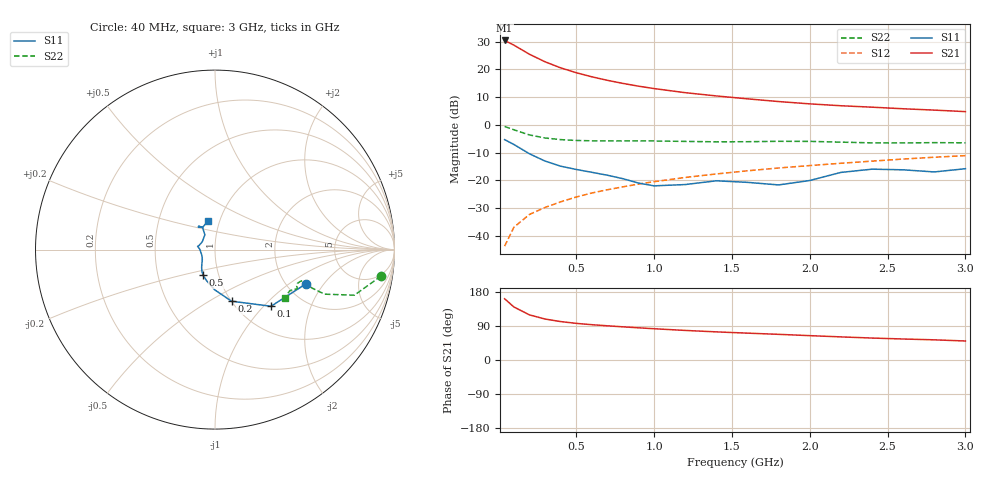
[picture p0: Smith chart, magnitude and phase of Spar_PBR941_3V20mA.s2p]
! Filename:  PBR941G.S2P  Version:  3.0
! NXP part #:  PBR941  Date: July 1998
! Bias condition:  Vce=3V, Ic=20mA
#  MHz  S  MA  R 50
! Freq  S11  S21  S12  S22
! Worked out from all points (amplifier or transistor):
!   21 points, 40 MHz to 3 GHz, reference 50 ohm
!   highest |S21| = 30.4 dB at 40 MHz (marker M1)
!   |S21| within 3 dB of that: start of sweep to 139.8 MHz
!   unconditionally stable (mu >= 1): 651.9 MHz to 2.236 GHz
!   at 300 MHz: K = 0.87, MSG = 26.2 dB, |S12| = -29.7 dB
!   at 1 GHz: K = 1.03, MAG = 15.7 dB, |S12| = -20.4 dB
!   at 3 GHz: K = 0.97, MSG = 7.9 dB, |S12| = -11.1 dB
!   S11 on the Smith chart (normalised r, x): 40 MHz: 2.55, -1.37; 100 MHz: 1.40, -1.10; 200 MHz: 1.00, -0.63; 500 MHz: 0.84, -0.25; 3 GHz: 0.88, +0.29
40  0.5433 -20.4  33.04 161.6  0.006582 81.4  0.9368 -9.1
100  0.444 -45.3  27.18 139.8  0.01444 74.7  0.8169 -18.1
200  0.3019 -72.3  18.64 119.0  0.02453 72.3  0.6591 -22.1
300  0.2233 -90.7  13.64 108.1  0.03277 74.9  0.5815 -21.6
400  0.181 -104.5  10.63 101.4  0.04127 76.0  0.5437 -20.7
500  0.1578 -114.9  8.688 96.7  0.05041 77.5  0.5252 -20.1
600  0.1404 -121.3  7.333 93.2  0.05953 78.1  0.5172 -19.8
700  0.1244 -126.7  6.342 90.2  0.06809 78.9  0.5151 -19.7
800  0.1077 -132.7  5.577 87.5  0.07686 79.3  0.5156 -19.6
900  0.0899 -142.0  4.975 85.0  0.08615 79.5  0.5151 -19.7
1000  0.08006 -155.2  4.504 82.5  0.0952 79.5  0.5138 -19.9
1200  0.08452 178.8  3.799 78.0  0.1133 79.3  0.5049 -20.7
1400  0.09872 169.3  3.319 74.2  0.1311 79.0  0.4961 -22.4
1600  0.09256 166.4  2.943 70.9  0.1494 78.8  0.4984 -24.1
1800  0.0832 148.7  2.631 67.7  0.1678 78.4  0.5067 -25.2
2000  0.09993 124.4  2.39 64.3  0.1855 77.5  0.5052 -25.9
2200  0.1397 119.4  2.211 61.0  0.204 76.5  0.4896 -26.8
2400  0.1598 124.4  2.084 57.9  0.2229 75.7  0.4749 -29.1
2600  0.1556 127.0  1.951 55.4  0.2429 75.2  0.4735 -32.1
2800  0.1425 118.6  1.845 53.2  0.262 74.4  0.4795 -34.0
3000  0.1629 104.1  1.733 50.1  0.2799 73.2  0.4757 -34.6
